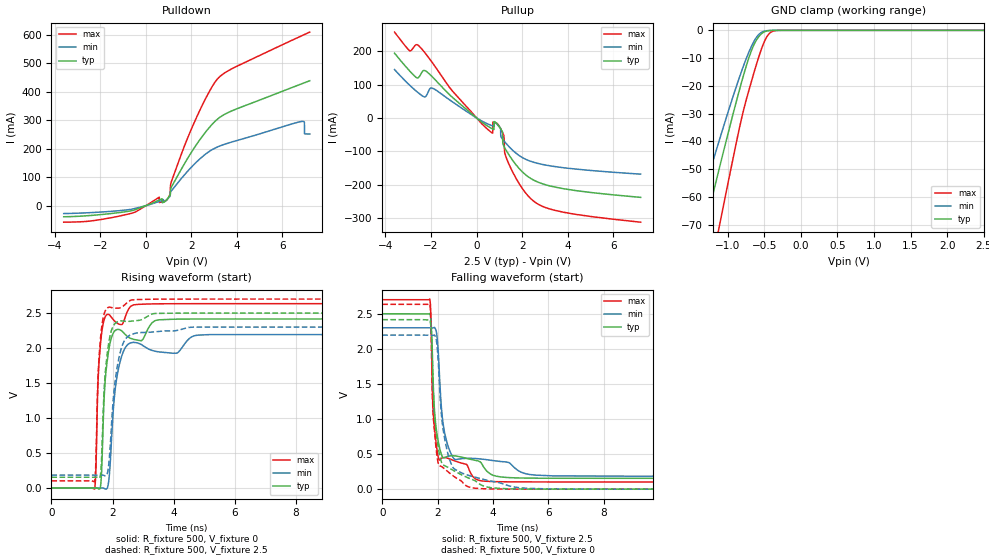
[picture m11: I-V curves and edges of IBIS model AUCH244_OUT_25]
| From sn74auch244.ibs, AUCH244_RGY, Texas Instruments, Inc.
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[Model]   AUCH244_OUT_25
Model_type  3-state
Enable   Active-Low
Vref =   0
Rref =   500
Cref =   30p
Vmeas =   1.25
| variable   typ   min   max
C_comp   5.46pF   4.91pF   5.71pF
| C_pullup   8.04pF   4.36pF   12.23pF
| C_pulldown   6.91pF   4.95pF   15.53pF
| C_tri-state   5.46pF   4.91pF   5.71pF
[Temperature Range]   40   100   -40
| Ambient temperature   25   85   -40
[Voltage range]   2.5   2.3   2.7
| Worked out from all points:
|   slope of the pulldown table from 0 to 0.375 V, typ, clamps not added: 30.7 ohm
|   slope of the pullup table from 0 to 0.375 V, typ, clamps not added: 19.3 ohm
|   GND clamp passes 1 mA (typ) near -0.53 V on its own axis
|   rising waveform, R_fixture 500, V_fixture 0: 20-80 % time 200ps typ, 285ps min, 146ps max; typ from 0 V to 2.42 V
|   falling waveform, R_fixture 500, V_fixture 2.5: 20-80 % time 249ps typ, 348ps min, 182ps max; typ from 2.5 V to 0.154 V
|   rising waveform, R_fixture 500, V_fixture 2.5: 20-80 % time 202ps typ, 293ps min, 147ps max; typ from 0.154 V to 2.5 V
|   falling waveform, R_fixture 500, V_fixture 0: 20-80 % time 272ps typ, 386ps min, 187ps max; typ from 2.42 V to 0 V
[GND Clamp]
| AUCH244_OUT_25
|   Voltage   I(typ)   I(min)   I(max)
-3.6V     -322.8mA   -271.3mA   -392.8mA
-1.46V    -86.94mA   -70.17mA   -115.9mA
-1.295V   -69.04mA   -55.4mA    -94.3mA
-1.105V   -48.71mA   -38.78mA   -69.36mA
-850mV    -22.51mA   -17.75mA   -36.48mA
-785mV    -16.32mA   -12.88mA   -28.97mA
-725mV    -11.06mA   -8.766mA   -23.02mA
-625mV    -4.338mA   -3.266mA   -13.84mA
-520mV    -878.8uA   -490.9uA   -5.429mA
-430mV    -104.5uA   -60.63uA   -1.111mA
-325mV    -4.915uA   -5.535uA   -43.94uA
2.5V      1.045nA    235.5nA    1.469nA
[Pulldown]
| AUCH244_OUT_25
|   Voltage   I(typ)   I(min)   I(max)
-3.6V     -38.75mA   -27.46mA   -57.79mA
-1.145V   -23.84mA   -17.22mA   -36.09mA
590mV     19.92mA    14.98mA    30.03mA
600mV     20.28mA    15.25mA    11.17mA
910mV     20.16mA    20.33mA    19.24mA
1.07V     37.88mA    45.66mA    41.07mA
1.915V    176.4mA    127.8mA    252.5mA
3.135V    303.2mA    205.9mA    444mA
6.825V    427.7mA    295.8mA    596.2mA
6.965V    431.9mA    293mA      601.3mA
6.97V     432.1mA    252.7mA    601.5mA
7.2V      439mA      251.9mA    609.9mA
[Pullup]
| AUCH244_OUT_25
|   Voltage   I(typ)   I(min)   I(max)
-3.6V     193.7mA    144.6mA    256.9mA
-2.935V   140.5mA    97.95mA    200.9mA
-2.49V    125.8mA    71.54mA    212.7mA
-1.91V    120.8mA    88.21mA    162.4mA
445mV     -22.7mA    -16.54mA   -31.6mA
945mV     -21.66mA   -22.17mA   -19.44mA
1.14V     -42.3mA    -63.2mA    -44.05mA
1.19V     -83.17mA   -67.47mA   -51.41mA
1.235V    -89.46mA   -71.21mA   -103.5mA
1.455V    -114mA     -88.07mA   -143.4mA
2.515V    -186.4mA   -132.8mA   -249.5mA
7.2V      -237.7mA   -168.2mA   -311.9mA
[Ramp]
| AUCH244_OUT_25
| variable   typ   min   max
dV/dt_r   1.46/2.00E-10   1.33/2.88E-10   1.59/1.47E-10
dV/dt_f   1.41/2.51E-10   1.27/3.49E-10   1.56/1.83E-10
R_load = 500
[Rising Waveform]
| AUCH244_OUT_25
R_fixture =   500
C_fixture =   0
L_fixture =   0
V_fixture =   0
V_fixture_min = 0
V_fixture_max = 0
|   Time   V(typ)   V(min)   V(max)
0s        13.61nV    40.86nV    2.147nV
1.415ns   533.5uV    13.11uV    -16.08mV
1.565ns   -15.99mV   694.2uV    1.828V
1.63ns    129mV      1.561mV    2.156V
1.73ns    1.319V     -6.895mV   2.41V
1.835ns   1.844V     4.247mV    2.481V
2.155ns   2.266V     1.612V     2.356V
2.69ns    2.124V     2.082V     2.617V
3.985ns   2.412V     1.926V     2.633V
34.99ns   2.416V     2.195V     2.634V
[Falling Waveform]
| AUCH244_OUT_25
R_fixture =   500
C_fixture =   0
L_fixture =   0
V_fixture =   2.5
V_fixture_min = 2.3
V_fixture_max = 2.7
|   Time   V(typ)   V(min)   V(max)
0s        2.5V       2.3V       2.7V
1.715ns   2.502V     2.299V     2.709V
1.76ns    2.394V     2.298V     2.413V
1.835ns   1.581V     2.298V     1.14V
1.9ns     1.043V     2.3V       823.9mV
2.035ns   653.9mV    1.87V      435.6mV
2.18ns    454mV      984.6mV    449.1mV
2.445ns   474.6mV    538mV      429mV
3.525ns   391.2mV    431.5mV    122.9mV
34.99ns   154.5mV    184.4mV    102.7mV
[Rising Waveform]
| AUCH244_OUT_25
R_fixture =   500
C_fixture =   0
L_fixture =   0
V_fixture =   2.5
V_fixture_min = 2.3
V_fixture_max = 2.7
|   Time   V(typ)   V(min)   V(max)
0s        154.5mV    184.4mV    102.6mV
1.415ns   155mV      184.4mV    88.56mV
1.525ns   149.2mV    184.6mV    1.579V
1.605ns   181.5mV    185.5mV    2.125V
1.69ns    1.024V     184.5mV    2.422V
1.845ns   1.977V     235.2mV    2.577V
1.955ns   2.237V     812.4mV    2.579V
2.21ns    2.383V     1.859V     2.571V
2.62ns    2.384V     2.195V     2.687V
34.99ns   2.5V       2.3V       2.7V
[Falling Waveform]
| AUCH244_OUT_25
R_fixture =   500
C_fixture =   0
L_fixture =   0
V_fixture =   0
V_fixture_min = 0
V_fixture_max = 0
|   Time   V(typ)   V(min)   V(max)
0s        2.416V     2.195V     2.634V
1.715ns   2.415V     2.194V     2.642V
1.755ns   2.32V      2.193V     2.405V
1.83ns    1.546V     2.191V     1.134V
1.895ns   1.01V      2.192V     786.4mV
2.02ns    598.7mV    1.833V     370.6mV
2.16ns    362mV      967.3mV    317.2mV
2.4ns     304.9mV    461.4mV    239.4mV
3.225ns   141.4mV    184mV      20.12mV
34.99ns   30.13uV    991.9nV    13.44uV
